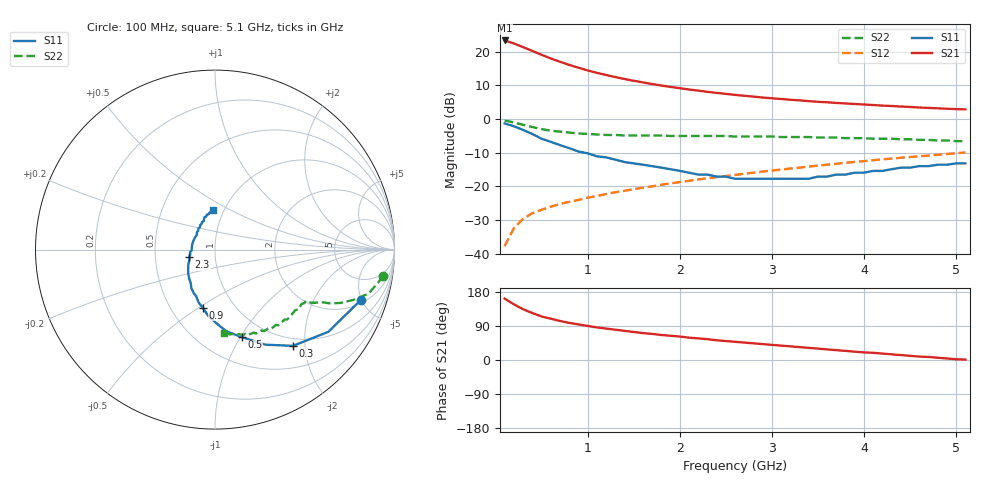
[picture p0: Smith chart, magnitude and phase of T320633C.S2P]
!AT-32063
!S AND NOISE PARAMETERS per side at Vce=2.7 V  Ic=5mA.  LAST UPDATED 11-11-96
# ghz s ma r 50
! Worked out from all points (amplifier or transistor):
!   51 points, 100 MHz to 5.1 GHz, reference 50 ohm
!   highest |S21| = 23.3 dB at 100 MHz (marker M1)
!   |S21| within 3 dB of that: start of sweep to 391 MHz
!   unconditionally stable (mu >= 1): 1.13 GHz to 4.294 GHz
!   at 900 MHz: K = 0.91, MSG = 19.6 dB, |S12| = -24.0 dB
!   at 2.6 GHz: K = 1.13, MAG = 9.7 dB, |S12| = -16.6 dB
!   at 5.1 GHz: K = 0.96, MSG = 6.4 dB, |S12| = -9.9 dB
!   lowest NFmin = 0.98 dB at 900 MHz
!   S11 on the Smith chart (normalised r, x): 100 MHz: 2.30, -4.94; 300 MHz: 0.86, -1.76; 500 MHz: 0.77, -1.01; 900 MHz: 0.72, -0.52; 2.3 GHz: 0.75, -0.06; 5.1 GHz: 0.89, +0.41
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0.1  0.86 -19.0  14.62 162.0  0.013 79.0  0.95 -9.0
0.2  0.78 -36.0  13.2 147.0  0.024 71.0  0.89 -16.0
0.3  0.69 -51.0  11.65 134.0  0.033 65.0  0.82 -20.0
0.4  0.6 -62.0  10.23 124.0  0.04 61.0  0.76 -23.0
0.5  0.51 -73.0  8.97 115.0  0.045 59.0  0.71 -25.0
0.6  0.46 -82.0  7.91 109.0  0.05 58.0  0.67 -26.0
0.7  0.41 -89.0  7.07 103.0  0.055 57.0  0.65 -27.0
0.8  0.37 -96.0  6.35 98.0  0.059 57.0  0.63 -28.0
0.9  0.33 -102.0  5.77 94.0  0.063 57.0  0.61 -29.0
1  0.31 -107.0  5.26 90.0  0.068 58.0  0.6 -29.0
1.1  0.28 -112.0  4.84 86.0  0.072 57.0  0.59 -30.0
1.3  0.25 -122.0  4.19 80.0  0.082 58.0  0.58 -31.0
1.4  0.23 -126.0  3.92 77.0  0.086 58.0  0.57 -32.0
1.6  0.21 -134.0  3.49 71.0  0.096 58.0  0.57 -34.0
1.8  0.19 -142.0  3.14 66.0  0.106 57.0  0.57 -36.0
2.1  0.16 -155.0  2.74 59.0  0.121 56.0  0.56 -39.0
2.3  0.15 -164.0  2.53 55.0  0.132 56.0  0.56 -42.0
2.6  0.13 -178.0  2.28 48.0  0.148 54.0  0.55 -45.0
2.9  0.13 166.0  2.08 42.0  0.166 52.0  0.55 -49.0
3.5  0.14 136.0  1.8 30.0  0.204 48.0  0.53 -56.0
4.3  0.18 110.0  1.56 15.0  0.259 40.0  0.51 -69.0
5.1  0.22 93.0  1.39 1.0  0.319 32.0  0.47 -84.0
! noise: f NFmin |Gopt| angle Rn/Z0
0.9  0.98  0.45  51  0.23
1.8  1.5  0.29  100  0.16
2.4  1.77  0.33  153  0.11
